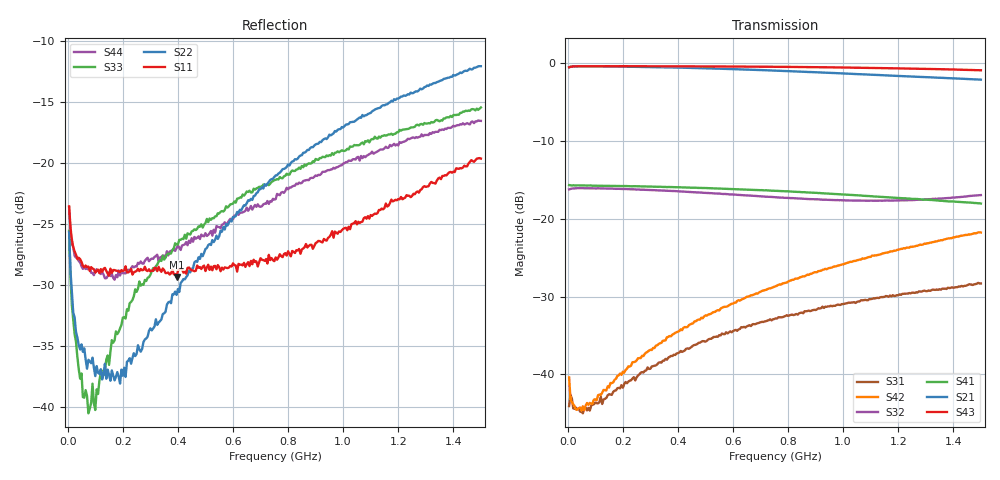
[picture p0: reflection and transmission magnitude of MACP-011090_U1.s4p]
!Agilent Technologies,E5071C,MY46110647,A.11.31
!Date: Tue Jan 18 13:56:48 2022 DD
!Data & Calibration Information:
!MACP-011090 soldered onto PT-0003645 with F connectors, Port1 (pin1) Port2 (pin6) Port3 (pin4) Port4 (pin3)
!Freq	S11:SOLT4(ON)	S12:SOLT4(ON)	S13:SOLT4(ON)	S14:SOLT4(ON)
!	S21:SOLT4(ON)	S22:SOLT4(ON)	S23:SOLT4(ON)	S24:SOLT4(ON)
!	S31:SOLT4(ON)	S32:SOLT4(ON)	S33:SOLT4(ON)	S34:SOLT4(ON)
!	S41:SOLT4(ON)	S42:SOLT4(ON)	S43:SOLT4(ON)	S44:SOLT4(ON)
!PortZ  Port1:75+j0  Port2:75+j0  Port3:75+j0  Port4:75+j0
!Above PortZ is port z conversion or system Z0 setting when saving the data.
!When reading, reference impedance value at option line is always used.
# Hz S MA R 75
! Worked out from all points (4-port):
!   300 points, 5 MHz to 1.5 GHz, reference 75 ohm
!   strongest paths, dB at 5 MHz, 380 MHz, 755 MHz, 1.13 GHz, 1.5 GHz:
!     S43: -0.5, -0.4, -0.4, -0.6, -0.9
!     S21: -0.5, -0.5, -0.9, -1.5, -2.1
!     S41: -15.6, -15.9, -16.4, -17.1, -18.0
!     S32: -16.2, -16.4, -17.2, -17.7, -16.9
!     S42: -40.4, -34.9, -28.7, -24.6, -21.7
!     S31: -44.1, -37.6, -32.8, -30.2, -28.3
!   lowest |S11| = -29.4 dB at 395 MHz (marker M1), VSWR 1.07, Z = 72.6 + j4.41 ohm
!   |S11| at or under -10 dB: start of sweep to end of sweep
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5000000  0.06626 143.8  0.9479 2.2  0.01113 141.5  0.1645 -179.6
         0.9451 2.2  0.05214 121.6  0.1557 4.8  0.007879 143.7
         0.006257 140.9  0.1548 3.9  0.05257 123.1  0.9449 2.4
         0.1652 -179.9  0.009567 144.1  0.9445 2.4  0.06556 143.3
3e7  0.04193 156.2  0.9584 -0.5  0.005935 152.8  0.1643 177.5
     0.9584 -0.5  0.0202 130.6  0.1575 0.6  0.006168 175.2
     0.00611 150.5  0.1575 0.6  0.01844 145.0  0.9582 -0.2
     0.1643 177.4  0.005934 177.2  0.9586 -0.2  0.04085 164.0
7.5e7  0.03752 157.4  0.9592 -2.6  0.00614 140.6  0.164 173.5
       0.9597 -2.6  0.01556 127.2  0.1576 -1.0  0.007001 -167.7
       0.006099 142.1  0.1577 -0.9  0.009384 -168.7  0.9601 -2.0
       0.164 173.4  0.006376 -164.8  0.96 -1.9  0.03648 177.3
1.9e8  0.03559 147.9  0.955 -7.1  0.008093 114.0  0.1627 163.7
       0.9554 -7.1  0.01243 97.2  0.1561 -3.2  0.01005 -153.2
       0.008132 114.7  0.1562 -3.3  0.02095 -122.1  0.9595 -5.6
       0.1628 163.7  0.01013 -154.0  0.96 -5.6  0.03448 -161.2
3.95e8  0.03404 117.1  0.9414 -14.8  0.01357 83.0  0.16 146.7
        0.9412 -14.8  0.02872 33.0  0.151 -6.2  0.01869 -164.4
        0.01362 85.2  0.1508 -6.3  0.04619 -104.2  0.9579 -11.8
        0.1599 146.6  0.0187 -164.4  0.9578 -11.8  0.04458 -139.4
8.55e8  0.04453 40.1  0.8849 -31.0  0.02558 44.3  0.1489 109.1
        0.8842 -31.0  0.1099 -23.7  0.1354 -7.2  0.04146 149.1
        0.02473 45.0  0.135 -7.2  0.09592 -101.0  0.9476 -26.1
        0.1487 109.2  0.04272 149.3  0.9481 -26.0  0.08423 -121.4
1.5e9  0.1041 -41.5  0.7873 -51.0  0.04021 6.7  0.126 58.9
       0.7868 -50.9  0.2491 -66.6  0.1434 2.6  0.08075 85.4
       0.03848 7.6  0.1424 3.1  0.1686 -101.3  0.9016 -47.5
       0.1256 59.2  0.08184 86.5  0.9041 -47.5  0.1486 -128.4
